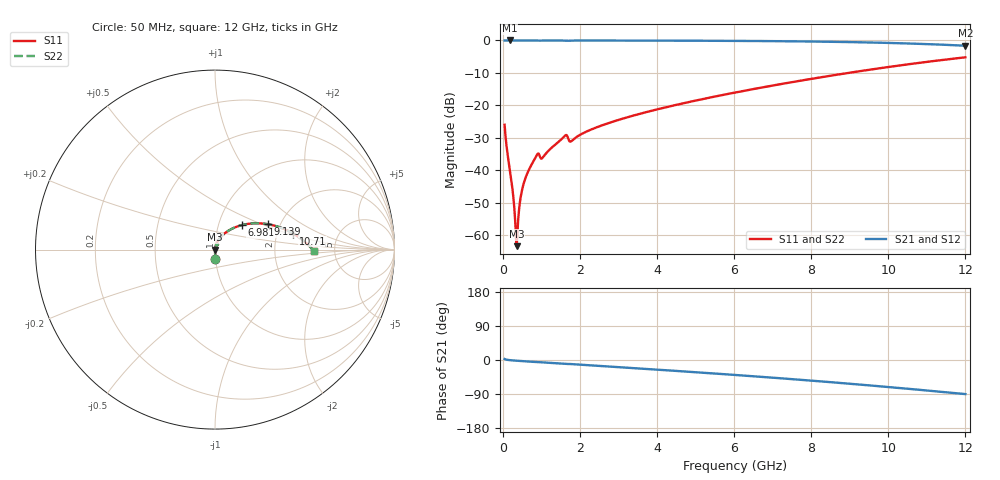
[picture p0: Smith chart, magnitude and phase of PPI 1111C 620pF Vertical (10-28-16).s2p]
# GHz S MA R 50
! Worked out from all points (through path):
!   1601 points, 50 MHz to 12 GHz, reference 50 ohm
!   highest |S21| = 0.00 dB at 177 MHz (marker M1); lowest = -1.6 dB at 12 GHz (marker M2)
!   group delay of S21, straight-line fit = 20.6 ps
!   lowest |S11| = -63.4 dB at 363.7 MHz (marker M3), VSWR 1.00, Z = 50.1 + j0.0111 ohm
!   |S11| at or under -10 dB: start of sweep to 8.968 GHz
!   |S22| runs from -63.4 to -5.2 dB; largest |S21 - S12| = 0
!   S11 on the Smith chart (normalised r, x): 50 MHz: 1.00, -0.10; 6.981 GHz: 1.29, +0.37; 9.139 GHz: 1.73, +0.55; 10.71 GHz: 2.45, +0.55; 12 GHz: 3.44, -0.05
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0.05  0.05025 -87.0  0.9984 2.6  0.9984 2.6  0.05025 -87.0
0.1769688  0.01103 -87.7  0.9994 -0.3  0.9994 -0.3  0.01103 -87.7
0.2516563  0.005272 -84.8  0.9994 -1.0  0.9994 -1.0  0.005272 -84.8
0.318875  0.001865 -71.9  0.9994 -1.6  0.9994 -1.6  0.001865 -71.9
0.3636875  0.0006774 9.4  0.9993 -1.9  0.9993 -1.9  0.0006774 9.4
0.4010313  0.001692 63.6  0.9993 -2.2  0.9993 -2.2  0.001692 63.6
0.46825  0.003906 76.3  0.9992 -2.7  0.9992 -2.7  0.003906 76.3
0.5429375  0.006199 79.4  0.9991 -3.2  0.9991 -3.2  0.006199 79.4
0.6624375  0.009668 80.5  0.999 -4.0  0.999 -4.0  0.009668 80.5
0.8715625  0.0166 76.1  0.9974 -5.5  0.9974 -5.5  0.0166 76.1
1.043344  0.01584 73.4  0.997 -6.3  0.997 -6.3  0.01584 73.4
1.610969  0.03391 70.9  0.9941 -10.3  0.9941 -10.3  0.03391 70.9
1.775281  0.02793 68.4  0.9942 -10.8  0.9942 -10.8  0.02793 68.4
2.044156  0.03616 74.2  0.9972 -12.6  0.9972 -12.6  0.03616 74.2
4.038312  0.08765 62.9  0.9938 -25.7  0.9938 -25.7  0.08765 62.9
6.025  0.1574 49.6  0.9844 -39.4  0.9844 -39.4  0.1574 49.6
6.981  0.2009 42.6  0.9761 -46.5  0.9761 -46.5  0.2009 42.6
8.019156  0.2568 34.7  0.9625 -54.6  0.9625 -54.6  0.2568 34.7
9.139469  0.3278 25.5  0.9402 -63.8  0.9402 -63.8  0.3278 25.5
10.01331  0.3905 17.9  0.9157 -71.4  0.9157 -71.4  0.3905 17.9
10.70791  0.4441 11.6  0.8906 -77.7  0.8906 -77.7  0.4441 11.6
12  0.5494 -0.5  0.8294 -90.0  0.8294 -90.0  0.5494 -0.5
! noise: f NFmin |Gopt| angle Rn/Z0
0.05  0.0003805  0.8688  0.2882  0.0006238
1.372  0.004653  0.7286  7.037  0.0034
2.701  0.006868  0.6563  13.66  0.003759
4.031  0.009088  0.6255  20.06  0.00441
5.36  0.01135  0.6125  26.24  0.005174
6.682  0.01366  0.6096  32.12  0.006015
8.012  0.01611  0.6141  37.77  0.00699
9.341  0.01876  0.6248  43.16  0.008157
10.67  0.02171  0.6408  48.31  0.009599
12  0.02507  0.6613  53.26  0.01143
